(* Logix 5000 DataType export Std_DiscreteInput; software revision 30.00 *)

TYPE AAStd_DiscreteAlarm :   // Discrete Alarm - Version 1.0 7/05/07 Modified 1/08 for Hills 10.6815 Added Alarm Reset Bit
STRUCT
   AckC : BOOL;   // ALARM ACKNOWLEDGE
   LatchA : BOOL;   // ALARM LATCH
   DetectS : BOOL;   // ALARM DETECT
   BitS : BOOL;   // ALARM MISCOMPARE
   InhibitC : BOOL;   // ALARM INHIBIT
   ResetC : BOOL;   // ALARM RESET
   Tmr : TIMER;   // ALARM Timer
END_STRUCT
END_TYPE

TYPE Std_DiscreteInput :   // Discrete Input - Version 1.0
STRUCT
   InI : BOOL;   // INPUT
   DisAlm : AAStd_DiscreteAlarm;   // DISCRETE ALARM
END_STRUCT
END_TYPE
